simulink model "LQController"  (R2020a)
settings: Solver=VariableStepAuto  StartTime=0.0  StopTime=10.0  RelTol=1e-3
InitFcn:
  | initParams
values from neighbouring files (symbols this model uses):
  K = 10    [initParams.m]
  ud = 0    [initParams.m]
  x0 = [0.2;0.1]    [initParams.m]
  xd = [pi;0]    [initParams.m]

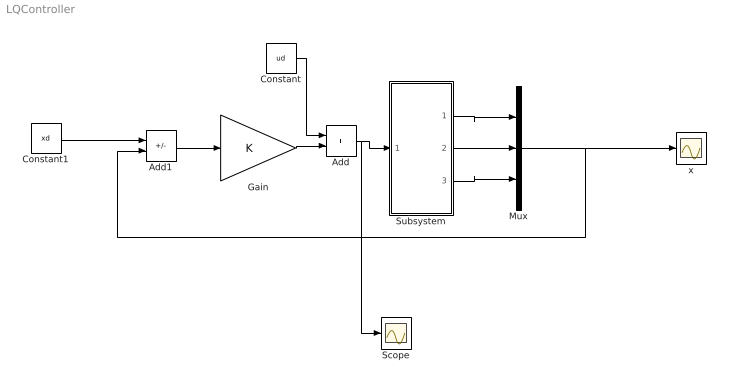
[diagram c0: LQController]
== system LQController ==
  Add : Sum
  Add1 : Sum  Inputs=+-
  Constant : Constant  Value=ud
  Constant1 : Constant  Value=xd
  Gain : Gain  Gain=K  Multiplication=Matrix(K*u) (u vector)
  Mux : Mux  Inputs=3
  Scope : Scope
  Subsystem : Subsystem
  x : Scope
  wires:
  Subsystem/2(x2) -> Mux/2
  Subsystem/1(x1) -> Mux/1
  Subsystem/3(x3) -> Mux/3
  Mux/1 -> Add1/2, x/1
  Gain/1 -> Add/2
  Add/1 -> Scope/1, Subsystem/1(u)
  Constant/1 -> Add/1
  Add1/1 -> Gain/1
  Constant1/1 -> Add1/1

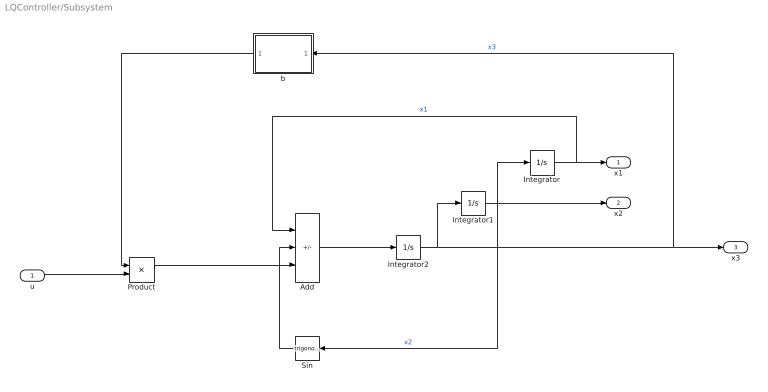
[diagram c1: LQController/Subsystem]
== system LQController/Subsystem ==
  u : Inport
  Add : Sum  Inputs=--+
  Integrator : Integrator  InitialCondition=x0(1)
  Integrator1 : Integrator  InitialCondition=x0(2)
  Integrator2 : Integrator  InitialCondition=x0(3)
  Product : Product
  Sin : Trigonometry
  b : MATLAB Function  TreatAsAtomicUnit=on
  x1 : Outport
  x2 : Outport  Port=2
  x3 : Outport  Port=3
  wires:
  Integrator/1 -> Add/1, x1/1  "x1"
  Sin/1 -> Add/2
  Integrator1/1 -> x2/1, Sin/1, Integrator/1  "x2"
  u/1 -> Product/2
  Integrator2/1 -> b/1(x3), x3/1, Integrator1/1  "x3"
  Add/1 -> Integrator2/1
  Product/1 -> Add/3
  b/1(y) -> Product/1

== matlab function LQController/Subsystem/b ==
function y = fcn(x3)

y = exp(-x3)+1;
